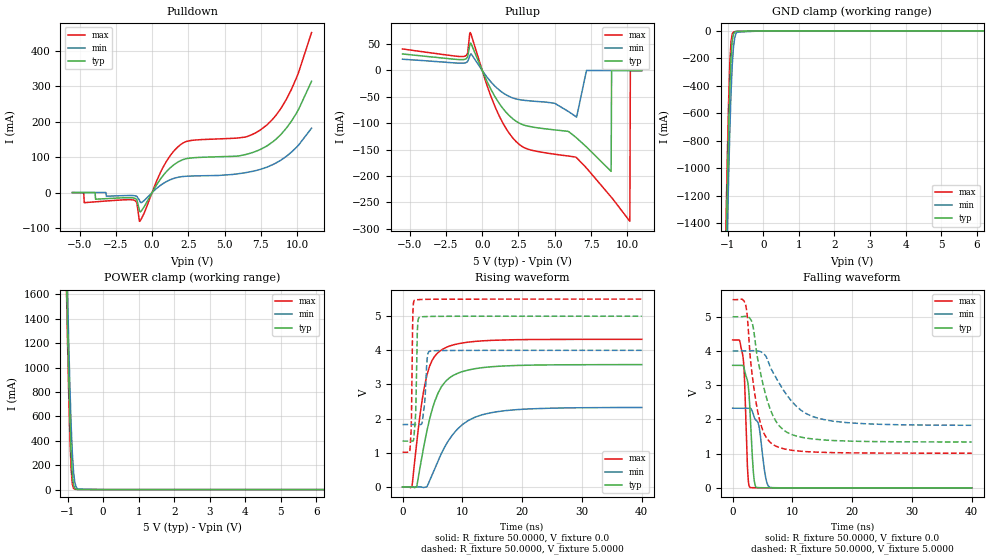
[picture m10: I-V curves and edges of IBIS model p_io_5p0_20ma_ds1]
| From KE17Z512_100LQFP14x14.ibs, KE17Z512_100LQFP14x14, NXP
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[Model] p_io_5p0_20ma_ds1
|   Model p_io_5p0_20ma_ds1
| This model was characterised for following simulation conditions:
| External (pad) voltage:
|   - Typ: 5.0V,   - Min: 4.0V,   - Max: 5.5V
| Library cells for typ/min/max conditions are connected as defined below:
|  pad - External Pad
|  ipp_do_lv - Core Input
|  ipp_obe_lv - Output Buffer Enable
|  abt_close_nor_rst_mv - vdde
|  dvdd - dvdd
|  dvss - dvss
|  esd_boost - vdde
|  ipp_dse_lv - dvdd
|  ipp_ina_280_mv - NC
|  ipp_ina_40_a_mv - NC
|  ipp_ina_40_b_mv - NC
|  ipp_ina_40_c_mv - NC
|  ipp_ina_40_d_mv - NC
|  ipp_ina_40_e_mv - NC
|  ipp_ina_40_f_mv - NC
|  ipp_ina_40_g_mv - NC
|  ipp_ina_40_h_mv - NC
|  ipp_ind_lv - NC
|  vdde - vdde
|  vsse - vsse
| All other pins connected to ground
Model_type I/O
Polarity   Non-Inverting
Enable   Active-High
Vinl =   1.5000V
Vinh =   3.5000V
Vmeas =  2.5000V
Cref =   50.0000F
C_comp   2.8015pF   2.6791pF   2.9922pF
[Model Spec]
| variable   typ   min   max
Vinh   3.5000V   2.8000V   3.8500V
Vinl   1.5000V   1.2000V   1.6500V
S_overshoot_high   5.3000V   4.3000V   5.8000V
S_overshoot_low   -0.3000V   -0.3000V   -0.3000V
Vmeas   2.5000V   2.0000V   2.7500V
[Temperature Range]   25.0000   0.1250k   -40.0000
[Voltage Range]   5.0000V   4.0000V   5.5000V
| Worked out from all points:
|   slope of the pulldown table from 0 to 0.75 V, typ, clamps not added: 15.7 ohm
|   slope of the pullup table from 0 to 0.75 V, typ, clamps not added: 17.4 ohm
|   rising waveform, R_fixture 50.0000, V_fixture 0.0: 20-80 % time 3.22ns typ, 5.09ns min, 2.28ns max; typ from 0 V to 3.58 V
|   rising waveform, R_fixture 50.0000, V_fixture 5.0000: 20-80 % time 260ps typ, 483ps min, 195ps max; typ from 1.34 V to 5 V
|   falling waveform, R_fixture 50.0000, V_fixture 0.0: 20-80 % time 682ps typ, 1.04ns min, 511ps max; typ from 3.58 V to 0 V
|   falling waveform, R_fixture 50.0000, V_fixture 5.0000: 20-80 % time 3.08ns typ, 5.24ns min, 1.99ns max; typ from 5 V to 1.34 V
[Pulldown]
|Voltage   I(typ)   I(min)   I(max)
-5.5V     -40uA      10uA       -280uA
-4.718V   -30uA      10uA       -460uA
-4.684V   -30uA      10uA       -28.62mA
-1.216V   -15.84mA   -8.966mA   -22.1mA
-1.046V   -21.21mA   -11.16mA   -30.99mA
-842mV    -54.16mA   -24.86mA   -81.17mA
722mV     46.26mA    24.51mA    68.8mA
1.98V     90.4mA     44.6mA     135.9mA
6.468V    107.7mA    56.4mA     157.4mA
8.338V    143.7mA    79.2mA     208.3mA
9.596V    200.8mA    113.7mA    290.4mA
11V       314.5mA    182mA      452.3mA
[Pullup]
|Voltage   I(typ)   I(min)   I(max)
-5.5V     31.4mA     21.4mA     40.8mA
-1.24V    20.94mA    14.13mA    26.83mA
-832mV    51.4mA     29.6mA     71.88mA
868mV     -49.09mA   -29.51mA   -67.74mA
2.194V    -93.34mA   -52.79mA   -130.6mA
6.512V    -127.9mA   -88.28mA   -165.4mA
7.192V    -144.9mA   -20uA      -184.8mA
8.892V    -191.2mA   10uA       -239.7mA
8.926V    -90uA      10uA       -240.8mA
10.18V    -30uA      0A         -285.8mA
10.22V    -30uA      -10uA      -390uA
11V       -60uA      0A         -270uA
[GND_clamp]
|Voltage   I(typ)   I(min)   I(max)
-5.5V     -74.62A    -74.49A    -74.76A
-1.08V    -1.983A    -2.319A    -1.787A
-1.046V   -1.53A     -1.877A    -1.323A
-1.012V   -1.108A    -1.459A    -893.4mA
-978mV    -729.3mA   -1.075A    -519.1mA
-944mV    -416.7mA   -736.6mA   -235.7mA
-910mV    -195.2mA   -457.3mA   -77.19mA
-876mV    -73.87mA   -251.2mA   -21.92mA
-842mV    -25.05mA   -121.5mA   -8.825mA
-740mV    -3.106mA   -9.724mA   -4.306mA
0V        -97.39pA   -840.9pA   -997.7pA
11V       0A         0A         0A
[POWER_clamp]
|Voltage   I(typ)   I(min)   I(max)
-5.5V     79A        78.7A      79.25A
-1.036V   1.833A     2.072A     1.706A
-1.002V   1.371A     1.626A     1.227A
-968mV    946.6mA    1.212A     789.9mA
-934mV    579.8mA    842.9mA    422.7mA
-900mV    297mA      533.2mA    167mA
-866mV    120.4mA    298.4mA    45.78mA
-832mV    39.59mA    145.6mA    10.75mA
-798mV    11.97mA    63.04mA    3.299mA
-696mV    1.006mA    4.196mA    1.128mA
0V        141.3pA    3.127nA    117.5pA
11V       0A         0A         0A
[Ramp]
| variable   typ   min   max
dV/dt_r  2.1488/3.2243n   1.3956/5.0857n   2.5937/2.2802n
dV/dt_f  2.1952/3.0796n   1.3030/5.2438n   2.6923/1.9876n
R_load = 50.0000
[Rising Waveform]
R_fixture= 50.0000
V_fixture= 0.0
V_fixture_min= 0.0
V_fixture_max= 0.0
|time   V(typ)   V(min)   V(max)
0s        988.8pV    11.54nV    7.472nV
1.581ns   195.2uV    5.908uV    18.82mV
2.37ns    17.29mV    7.635uV    1.294V
3.251ns   889.5mV    -7.559mV   2.511V
4.004ns   1.581V     -1.939mV   3.229V
5.318ns   2.473V     508.6mV    3.811V
6.667ns   2.973V     1.038V     4.029V
10.11ns   3.382V     1.839V     4.219V
14.48ns   3.513V     2.162V     4.289V
40ns      3.581V     2.326V     4.323V
[Rising Waveform]
R_fixture= 50.0000
V_fixture= 5.0000
V_fixture_min= 4.0000
V_fixture_max= 5.5000
|time   V(typ)   V(min)   V(max)
0s        1.341V     1.825V     1.013V
1.244ns   1.341V     1.825V     1.081V
1.475ns   1.341V     1.825V     1.858V
1.726ns   1.342V     1.825V     5.052V
1.976ns   1.641V     1.825V     5.467V
2.199ns   2.187V     1.825V     5.479V
2.508ns   4.684V     1.825V     5.484V
2.833ns   4.971V     1.826V     5.488V
4.541ns   4.993V     3.974V     5.496V
40ns      5V         4V         5.5V
[Falling Waveform]
R_fixture= 50.0000
V_fixture= 0.0
V_fixture_min= 0.0
V_fixture_max= 0.0
|time   V(typ)   V(min)   V(max)
0s        3.582V     2.327V     4.323V
1.134ns   3.582V     2.327V     4.313V
1.751ns   3.573V     2.327V     3.798V
2.017ns   3.419V     2.327V     3.02V
2.542ns   3.072V     2.327V     383.1mV
2.879ns   2.329V     2.328V     16.02mV
3.468ns   448.8mV    2.134V     4.323mV
3.963ns   16.76mV    1.969V     2.679mV
6.238ns   1.565mV    15.63mV    803.2uV
40ns      786.1nV    6.619uV    -14.15uV
[Falling Waveform]
R_fixture= 50.0000
V_fixture= 5.0000
V_fixture_min= 4.0000
V_fixture_max= 5.5000
|time   V(typ)   V(min)   V(max)
0s        5V         4V         5.5V
2.137ns   5.011V     4V         5.375V
2.433ns   5.013V     4V         5.051V
3.247ns   4.842V     4.01V      3.332V
4.117ns   3.835V     4.006V     2.294V
5.269ns   2.891V     3.906V     1.581V
6.587ns   2.17V      3.425V     1.284V
10.43ns   1.526V     2.422V     1.088V
14.44ns   1.411V     2.028V     1.041V
40ns      1.341V     1.828V     1.013V
